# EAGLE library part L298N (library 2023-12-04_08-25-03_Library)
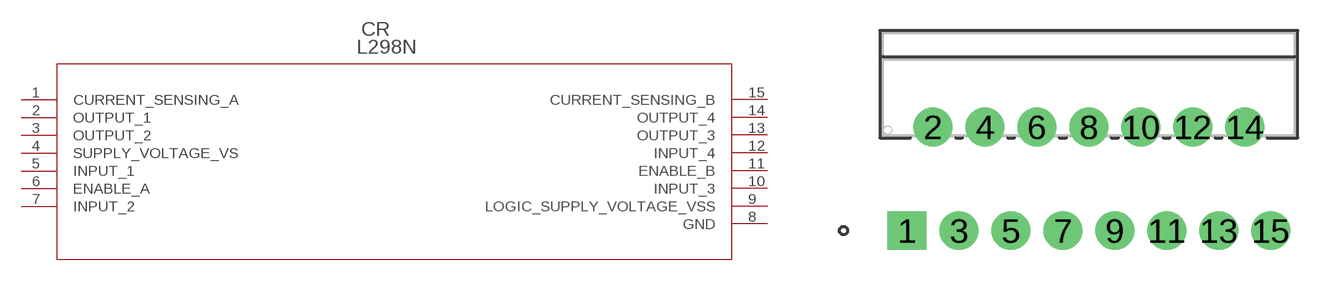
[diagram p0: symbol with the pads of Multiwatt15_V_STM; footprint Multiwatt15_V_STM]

Designator prefix CR

## L298NMultiwatt15_V_STM (Copyright: Copyright (C) 2023 Ultra Librarian. All rights reserved.; Manufacturer_Part_Number: L298N; Mfr_Name: STMicroelectronics)  [Multiwatt15_V_STM]
1  CURRENT_SENSING_A  in
2  OUTPUT_1  out
3  OUTPUT_2  out
4  SUPPLY_VOLTAGE_VS  pwr
5  INPUT_1  in
6  ENABLE_A  in
7  INPUT_2  in
8  GND  pas
9  LOGIC_SUPPLY_VOLTAGE_VSS  pwr
10  INPUT_3  in
11  ENABLE_B  in
12  INPUT_4  in
13  OUTPUT_3  out
14  OUTPUT_4  out
15  CURRENT_SENSING_B  in

## Footprint Multiwatt15_V_STM (pad centres in mm)
drill 1.27 pad 1.778 square: 1 0,0
drill 1.27 pad 1.778 round: 2 1.27,5.08; 3 2.54,0; 4 3.81,5.08; 5 5.08,0; 6 6.35,5.08; 7 7.62,0; 8 8.89,5.08; 9 10.16,0; 10 11.43,5.08; 11 12.7,0; 12 13.97,5.08; 13 15.24,0; 14 16.51,5.08; 15 17.78,0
